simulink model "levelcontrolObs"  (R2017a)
settings: Solver=ode3  StartTime=0.0  StopTime=10.0  FixedStep=0.1  RelTol=1e-3
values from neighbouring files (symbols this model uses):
  eta = 1e0    (= 1)    [levelcontrol_init3.m]    (also in levelcontrol_init4.m; levelcontrol_init5.m; levelcontrol_init6.m)
  h_est_init = 0.4    [levelcontrol_init3.m]    (also in levelcontrol_init4.m; levelcontrol_init5.m; levelcontrol_init6.m)
  h_init = 0.5    [levelcontrol_init3.m]    (also in levelcontrol_init4.m; levelcontrol_init5.m; levelcontrol_init6.m)
  h_set = 0.5    [ExamplePIbased.m]    (also in levelcontrol_init3.m; levelcontrol_init4.m; levelcontrol_init5.m; levelcontrol_init6.m)
  LEKF = [pEKF(1) pEKF(2); pEKF(2) pEKF(3)]*transpose(C)*REKFinv    [levelcontrol_init3.m]    (also in levelcontrol_init4.m; levelcontrol_init5.m; levelcontrol_init6.m)
  LLSO = eta*[pLSO(1) pLSO(2); pLSO(2) pLSO(3)]*transpose(C)*RLSOinv    [levelcontrol_init3.m]    (also in levelcontrol_init4.m; levelcontrol_init5.m; levelcontrol_init6.m)
  noise_ON = 0    [ExamplePIbased.m]    (also in levelcontrol_init3.m = 1; levelcontrol_init4.m; levelcontrol_init5.m; levelcontrol_init6.m = 1)
  Q = [1e-1 0; 0 1e0]    [levelcontrol_init3.m]    (also in levelcontrol_init4.m; levelcontrol_init5.m; levelcontrol_init6.m)
  q_in_est_init = 0.4    [levelcontrol_init3.m]    (also in levelcontrol_init4.m; levelcontrol_init5.m; levelcontrol_init6.m)
  sin_ON = 1    [ExamplePIbased.m]    (also in levelcontrol_init3.m; levelcontrol_init4.m = 0; levelcontrol_init5.m; levelcontrol_init6.m)
  t_delay = 2    [levelcontrol_init3.m]    (also in levelcontrol_init4.m; levelcontrol_init5.m; levelcontrol_init6.m)
  tau_c = 3    [ExamplePIbased.m]    (also in levelcontrol_init3.m; levelcontrol_init4.m; levelcontrol_init5.m; levelcontrol_init6.m)
  useEKF = 0    [levelcontrol_init3.m]    (also in levelcontrol_init4.m; levelcontrol_init5.m; levelcontrol_init6.m)
  useLSO = 1    [levelcontrol_init3.m]    (also in levelcontrol_init4.m; levelcontrol_init5.m; levelcontrol_init6.m)
undefined symbols (not defined in the file or in its folder): Riccati_init, Rinverse, roc
libraries: simulink x1

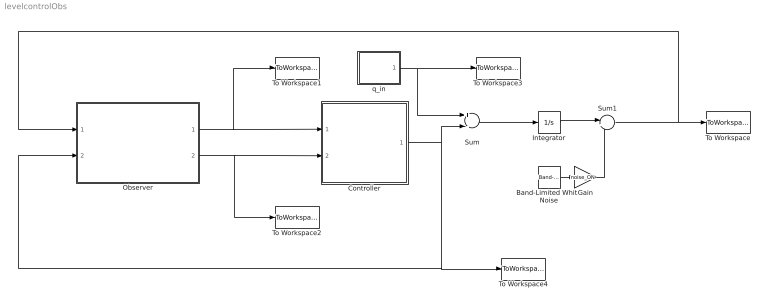
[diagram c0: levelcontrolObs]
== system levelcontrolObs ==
  Band-Limited White Noise : simulink/Sources/Band-Limited White Noise  Cov=noise_power  Ts=0.1  seed=[23341]
  Controller : Subsystem
  Gain : Gain  Gain=noise_ON
  Integrator : Integrator  InitialCondition=h_init
  Observer : Subsystem
  Sum : Sum  Inputs=+-
  Sum1 : Sum  Inputs=|++
  To Workspace : ToWorkspace  VariableName=h  SaveFormat=Structure With Time  SampleTime=-1
  To Workspace1 : ToWorkspace  VariableName=h_est  SaveFormat=Structure With Time  SampleTime=-1
  To Workspace2 : ToWorkspace  VariableName=q_in_est  SaveFormat=Structure With Time  SampleTime=-1
  To Workspace3 : ToWorkspace  VariableName=q_in  SaveFormat=Structure With Time  SampleTime=-1
  To Workspace4 : ToWorkspace  VariableName=q_out  SaveFormat=Structure With Time  SampleTime=-1
  q_in : Subsystem
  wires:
  q_in/1(q_in) -> To Workspace3/1, Sum/1
  Controller/1(q_out) -> Sum/2, Observer/2(q_out), To Workspace4/1
  Observer/2(q_in_est) -> Controller/2(q_in_est2), To Workspace2/1
  Observer/1(h_est) -> Controller/1(h_est), To Workspace1/1
  Sum/1 -> Integrator/1
  Integrator/1 -> Sum1/1
  Band-Limited White Noise/1 -> Gain/1
  Sum1/1 -> Observer/1(h), To Workspace/1
  Gain/1 -> Sum1/2

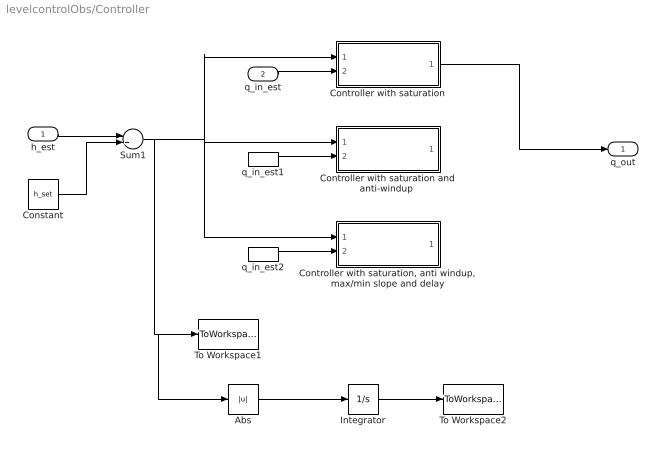
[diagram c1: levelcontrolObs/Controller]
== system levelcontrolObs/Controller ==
  h_est : Inport
  q_in_est : Inport  Port=2
  Abs : Abs
  Constant : Constant  Value=h_set
  Controller with saturation : Subsystem
  "Controller with saturation and anti-windup " : Subsystem  Commented=on
  "Controller with saturation, anti windup, max/min slope and delay" : Subsystem  Commented=on
  Integrator : Integrator
  Sum1 : Sum  Inputs=-+
  To Workspace1 : ToWorkspace  VariableName=error_level  SaveFormat=Structure With Time  SampleTime=-1
  To Workspace2 : ToWorkspace  VariableName=IAEObs  SaveFormat=Structure With Time  SampleTime=-1
  q_in_est1 : InportShadow  Port=2
  q_in_est2 : InportShadow  Port=2
  q_out : Outport
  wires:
  h_est/1 -> Sum1/1
  Sum1/1 -> Abs/1, To Workspace1/1, "Controller with saturation and anti-windup "/1(error_level), "Controller with saturation, anti windup, max/min slope and delay"/1(error_level), Controller with saturation/1(error_level)
  Constant/1 -> Sum1/2
  Controller with saturation/1(u) -> q_out/1
  q_in_est/1 -> Controller with saturation/2(q_in_est)
  q_in_est1/1 -> "Controller with saturation and anti-windup "/2(q_in_est)
  q_in_est2/1 -> "Controller with saturation, anti windup, max/min slope and delay"/2(q_in_est)
  Integrator/1 -> To Workspace2/1
  Abs/1 -> Integrator/1

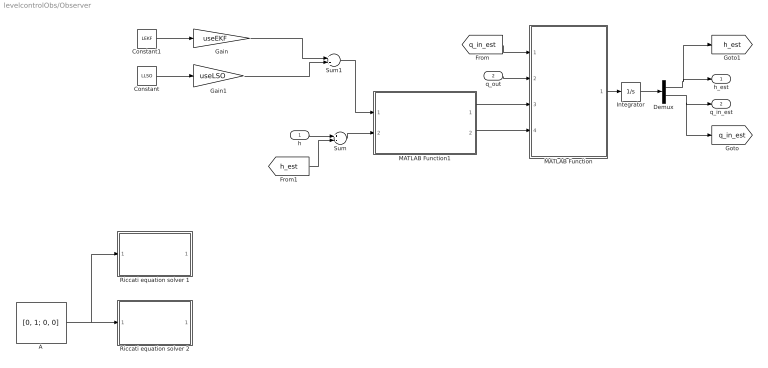
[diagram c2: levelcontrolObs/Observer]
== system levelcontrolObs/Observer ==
  h : Inport
  q_out : Inport  Port=2
  A : Constant  Commented=on  Value=[0, 1; 0, 0]
  Constant : Constant  Value=LLSO
  Constant1 : Constant  Value=LEKF
  Demux : Demux  Outputs=2
  Gain : Gain  Gain=useEKF
  Gain1 : Gain  Gain=useLSO
  Integrator : Integrator  InitialCondition=[h_est_init; q_in_est_init]
  MATLAB Function : MATLAB Function  TreatAsAtomicUnit=on
  MATLAB Function1 : MATLAB Function  TreatAsAtomicUnit=on
  Riccati equation solver 1 : Subsystem  Commented=on
  Riccati equation solver 2 : Subsystem  Commented=on
  Sum : Sum  Inputs=+-
  Sum1 : Sum
  h_est : Outport
  q_in_est : Outport  Port=2
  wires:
  A/1 -> Riccati equation solver 1/1(A), Riccati equation solver 2/1(A)
  h/1 -> Sum/1
  MATLAB Function/1(y) -> Integrator/1
  Integrator/1 -> Demux/1
  Demux/1 -> [h_est], h_est/1
  Demux/2 -> [q_in_est], q_in_est/1
  q_out/1 -> MATLAB Function/2(q_out)
  [q_in_est] -> MATLAB Function/1(q_in)
  [h_est] -> Sum/2
  MATLAB Function1/1(Compensation1) -> MATLAB Function/3(Compensation1)
  MATLAB Function1/2(Compensation2) -> MATLAB Function/4(Compensation2)
  Sum/1 -> MATLAB Function1/2(error_h)
  Sum1/1 -> MATLAB Function1/1(L)
  Constant1/1 -> Gain/1
  Constant/1 -> Gain1/1
  Gain1/1 -> Sum1/2
  Gain/1 -> Sum1/1

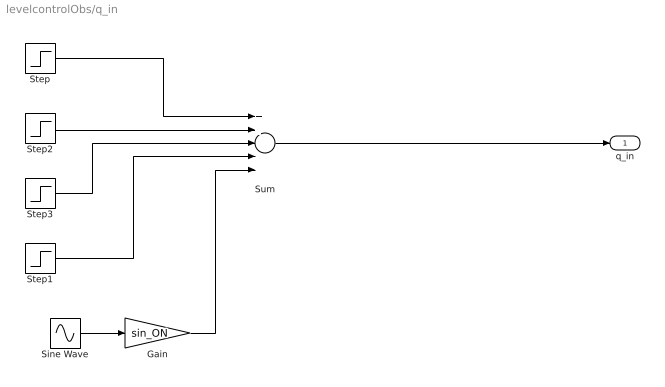
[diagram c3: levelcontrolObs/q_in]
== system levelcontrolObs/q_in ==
  Gain : Gain  Gain=sin_ON
  Sine Wave : Sin  Amplitude=0.05  SampleTime=0
  Step : Step  Time=20  Before=0.5  After=0.7  SampleTime=0
  Step1 : Step  Time=75  After=-0.9  SampleTime=0
  Step2 : Step  Time=40  After=0.2  SampleTime=0
  Step3 : Step  Time=60  After=0.1  SampleTime=0
  Sum : Sum  Inputs=5
  q_in : Outport
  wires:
  Sum/1 -> q_in/1
  Step/1 -> Sum/1
  Step1/1 -> Sum/4
  Sine Wave/1 -> Gain/1
  Gain/1 -> Sum/5
  Step2/1 -> Sum/2
  Step3/1 -> Sum/3

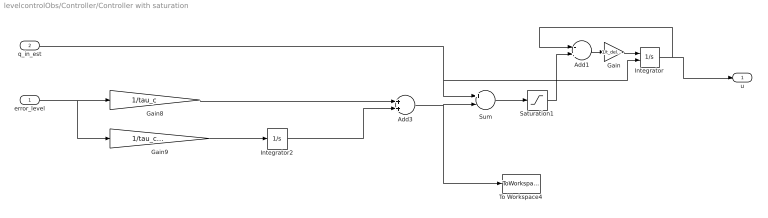
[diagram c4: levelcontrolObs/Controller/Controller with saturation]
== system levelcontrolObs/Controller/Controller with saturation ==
  error_level : Inport
  q_in_est : Inport  Port=2
  Add1 : Sum  Inputs=-+
  Add3 : Sum
  Gain : Gain  Gain=1/t_delay
  Gain8 : Gain  Gain=1/tau_c
  Gain9 : Gain  Gain=1/tau_c^2/4
  Integrator : Integrator  InitialConditionSource=external
  Integrator2 : Integrator  UpperSaturationLimit=100  LowerSaturationLimit=0
  Saturation1 : Saturate  UpperLimit=1  LowerLimit=0
  Sum : Sum  Inputs=+-
  To Workspace4 : ToWorkspace  VariableName=pi  SaveFormat=Structure With Time  SampleTime=-1
  u : Outport
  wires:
  Integrator2/1 -> Add3/2
  Gain9/1 -> Integrator2/1
  error_level/1 -> Gain9/1, Gain8/1
  Add3/1 -> To Workspace4/1, Sum/2
  Saturation1/1 -> Add1/2
  Gain8/1 -> Add3/1
  q_in_est/1 -> Sum/1, Integrator/2
  Sum/1 -> Saturation1/1
  Integrator/1 -> Add1/1, u/1
  Add1/1 -> Gain/1
  Gain/1 -> Integrator/1

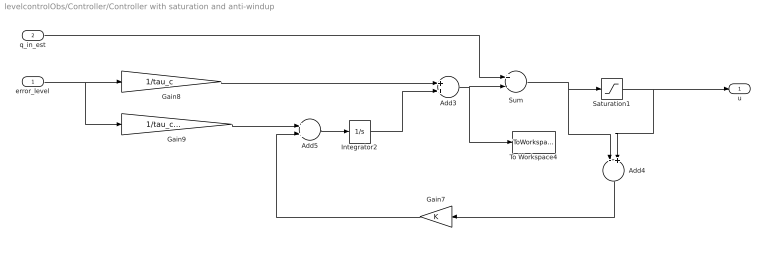
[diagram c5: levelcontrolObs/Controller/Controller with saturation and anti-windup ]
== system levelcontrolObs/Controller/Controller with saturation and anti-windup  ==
  error_level : Inport
  q_in_est : Inport  Port=2
  Add3 : Sum
  Add4 : Sum  Inputs=-+
  Add5 : Sum
  Gain7 : Gain
  Gain8 : Gain  Gain=1/tau_c
  Gain9 : Gain  Gain=1/tau_c^2/4
  Integrator2 : Integrator  UpperSaturationLimit=100  LowerSaturationLimit=0
  Saturation1 : Saturate  UpperLimit=1  LowerLimit=0
  Sum : Sum  Inputs=+-
  To Workspace4 : ToWorkspace  VariableName=pi  SaveFormat=Structure With Time  SampleTime=-1
  u : Outport
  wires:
  Integrator2/1 -> Add3/2
  Add5/1 -> Integrator2/1
  Add4/1 -> Gain7/1
  error_level/1 -> Gain9/1, Gain8/1
  Sum/1 -> Saturation1/1, Add4/1
  Gain9/1 -> Add5/1
  Saturation1/1 -> u/1, Add4/2
  Gain7/1 -> Add5/2
  Gain8/1 -> Add3/1
  q_in_est/1 -> Sum/1
  Add3/1 -> To Workspace4/1, Sum/2

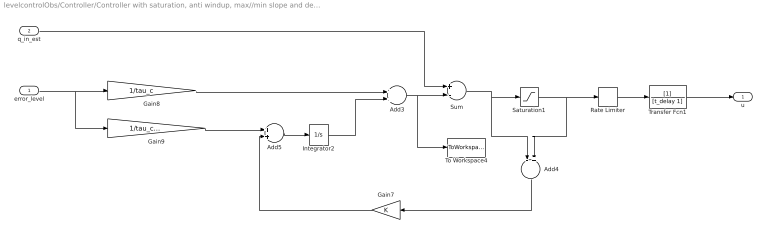
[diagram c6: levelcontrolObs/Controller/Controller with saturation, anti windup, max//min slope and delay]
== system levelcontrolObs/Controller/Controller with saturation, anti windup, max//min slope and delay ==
  error_level : Inport
  q_in_est : Inport  Port=2
  Add3 : Sum
  Add4 : Sum  Inputs=-+
  Add5 : Sum
  Gain7 : Gain
  Gain8 : Gain  Gain=1/tau_c
  Gain9 : Gain  Gain=1/tau_c^2/4
  Integrator2 : Integrator  InitialCondition=0.5  UpperSaturationLimit=100  LowerSaturationLimit=0
  Rate Limiter : RateLimiter  RisingSlewLimit=roc  FallingSlewLimit=-roc  SampleTimeMode=inherited
  Saturation1 : Saturate  UpperLimit=1  LowerLimit=0
  Sum : Sum  Inputs=+-
  To Workspace4 : ToWorkspace  VariableName=pi  SaveFormat=Structure With Time  SampleTime=-1
  Transfer Fcn1 : TransferFcn  Denominator=[t_delay 1]
  u : Outport
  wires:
  Integrator2/1 -> Add3/2
  Add5/1 -> Integrator2/1
  Add4/1 -> Gain7/1
  error_level/1 -> Gain9/1, Gain8/1
  Sum/1 -> Saturation1/1, Add4/1
  Gain9/1 -> Add5/1
  Saturation1/1 -> Add4/2, Rate Limiter/1
  Rate Limiter/1 -> Transfer Fcn1/1
  Transfer Fcn1/1 -> u/1
  Gain7/1 -> Add5/2
  Gain8/1 -> Add3/1
  q_in_est/1 -> Sum/1
  Add3/1 -> To Workspace4/1, Sum/2

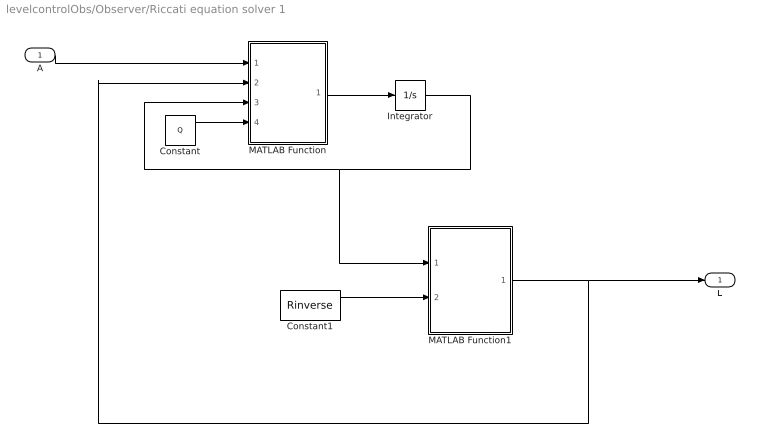
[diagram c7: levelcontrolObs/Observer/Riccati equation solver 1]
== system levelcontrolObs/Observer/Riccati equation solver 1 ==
  A : Inport
  Constant : Constant  Value=Q
  Constant1 : Constant  Value=Rinverse
  Integrator : Integrator  InitialCondition=Riccati_init
  MATLAB Function : MATLAB Function  TreatAsAtomicUnit=on
  MATLAB Function1 : MATLAB Function  TreatAsAtomicUnit=on
  L : Outport
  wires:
  A/1 -> MATLAB Function/1(A)
  MATLAB Function1/1(L) -> L/1, MATLAB Function/2(L)
  Constant/1 -> MATLAB Function/4(Q)
  Constant1/1 -> MATLAB Function1/2(R)
  MATLAB Function/1(dotP) -> Integrator/1
  Integrator/1 -> MATLAB Function1/1(P), MATLAB Function/3(P)

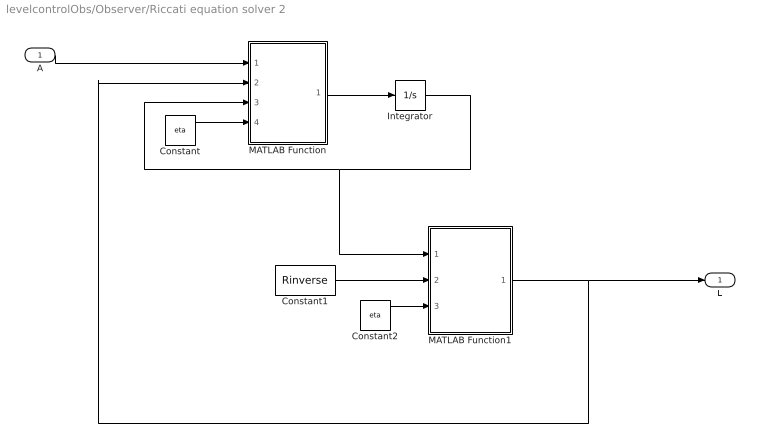
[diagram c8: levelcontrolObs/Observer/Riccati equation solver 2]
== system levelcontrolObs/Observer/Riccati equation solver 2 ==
  A : Inport
  Constant : Constant  Value=eta
  Constant1 : Constant  Value=Rinverse
  Constant2 : Constant  Value=eta
  Integrator : Integrator  InitialCondition=Riccati_init
  MATLAB Function : MATLAB Function  TreatAsAtomicUnit=on
  MATLAB Function1 : MATLAB Function  TreatAsAtomicUnit=on
  L : Outport
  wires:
  A/1 -> MATLAB Function/1(A)
  MATLAB Function1/1(L) -> L/1, MATLAB Function/2(L)
  Constant/1 -> MATLAB Function/4(eta)
  Constant1/1 -> MATLAB Function1/2(R)
  Constant2/1 -> MATLAB Function1/3(eta)
  MATLAB Function/1(dotP) -> Integrator/1
  Integrator/1 -> MATLAB Function1/1(P), MATLAB Function/3(P)

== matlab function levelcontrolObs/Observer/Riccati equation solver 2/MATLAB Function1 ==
function L = fcn(P,R,eta)

L = eta*P*[1; 0]*R;

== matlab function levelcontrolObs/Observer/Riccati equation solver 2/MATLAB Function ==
function dotP = fcn(A,L,P,eta)

dotP = eta*P+A*P+P*transpose(A) - L*[1 0]*P;

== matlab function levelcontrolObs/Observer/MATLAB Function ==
function y = fcn(q_in,q_out,Compensation1,Compensation2)

dh = (q_in - q_out) + Compensation1;

dq_in = Compensation2;

y = [dh; dq_in];

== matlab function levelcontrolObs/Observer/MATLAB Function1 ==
function [Compensation1,Compensation2] = fcn(L,error_h)

Compensation1 = L(1,:)*error_h;
Compensation2 = L(2,:)*error_h;

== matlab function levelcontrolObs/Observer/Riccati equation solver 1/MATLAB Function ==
function dotP = fcn(A,L,P,Q)

dotP = A*P+P*transpose(A) - L*[1 0]*P + Q;

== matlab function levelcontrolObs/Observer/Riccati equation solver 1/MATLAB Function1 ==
function L = fcn(P,R)

L = P*[1; 0]*R;
